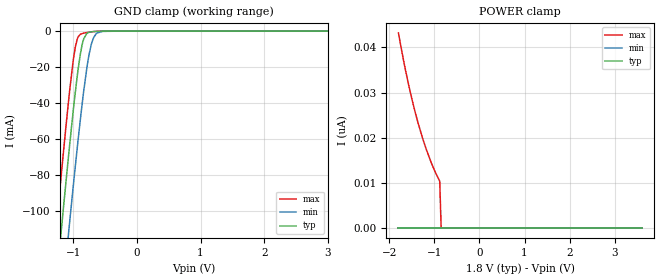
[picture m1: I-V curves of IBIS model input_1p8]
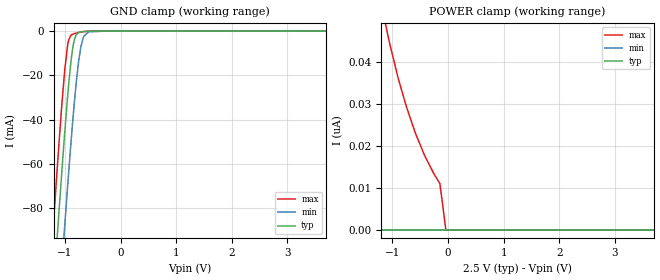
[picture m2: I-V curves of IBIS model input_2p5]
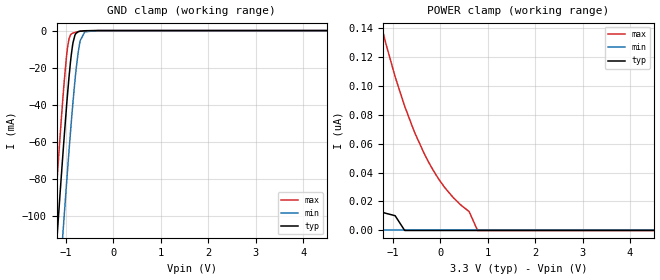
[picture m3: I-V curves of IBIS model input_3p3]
|Texas Instruments Incorporated
| Single Power Supply Single Buffer GATE with 3-State Output CMOS Logic
| Level Shifter
| Marketing part#   Digital Voltage Range   Package-type   #pins
| SN74LV4T125PWR   1.6V-5.5V   TSSOP   14
| SN74LV4T125RGYR   1.6V-5.5V   VQFN   14
[IBIS Ver]   4.1
[File name]   sn74lv4t125.ibs
[File Rev]   1.0
[Date]   3/20/2014
[Source]   Model built from TISPICE simulations at:
   Texas Instruments Incorporated.
   Analog-eLab, HPA
   12500 TI Blvd
   Dallas, TX -75243
   For Support e-mail: elab_ibis@list.ti.com
[Notes]   Revision History:
   Rev 1.0: 3/20/2014
   - Initial model based single channel device SN74LV1T125.
   - Model generated from simulations in TISPICE
   - Model matched to SPICE simulation
   - C_comp although listed in numerical order of value are
   obtained from varying PVT conditions. For PVT conditions for
   each specific value refer the buffer description under
   respective [Model]. IBIS model user is responsible for using
   appropriate C_comp to simulate for Signal Integrity.
[Disclaimer]
| This model is designed as an aid for customers of Texas Instruments.
| TI and its licensors and suppliers make no warranties, either expressed
| or implied, with respect to this  model, including the warranties of
| merchantability or fitness for a particular purpose. The model is
| provided solely on an "as is" basis. The entire risk as to its quality
| and performance is with the customer.
[Copyright]
(C) Copyright 2014 Texas Instruments Incorporated.All rights reserved.
|   SN74LV4T125PW
[Component]   SN74LV1T425PW
[Manufacturer]   TI
[Package]   |14 TSSOP  -  PW package
|   typ   min   max
R_pkg   0.19103   0.16967   0.21164
L_pkg   3.05250nH   2.65688nH   3.60685nH
C_pkg   0.48736pF   0.46092pF   0.53275pF
[Pin]  signal_name   model_name   R_pin   L_pin   C_pin
1   1OE   INPUT   0.19696   3.49379nH  0.52991pF
2   1A   INPUT   0.20002   3.01515nH  0.47995pF
3   1Y   OUTPUT   0.17897   2.78188nH  0.46369pF
4   2OE   INPUT   0.16967   2.65688nH  0.46092pF
5   2A   INPUT   0.17977   2.79132nH  0.46440pF
6   2Y   OUTPUT   0.19791   3.00095nH  0.47800pF
7   GND   GND   0.20476   3.55750nH  0.53043pF
8   3Y   OUTPUT   0.19575   3.49014nH  0.52950pF
9   3A   INPUT   0.20186   3.03224nH  0.48111pF
10   3OE   INPUT   0.18274   2.81298nH  0.46552pF
11   4Y   OUTPUT   0.17138   2.66909nH  0.46209pF
12   4A   INPUT   0.18361   2.81712nH  0.46577pF
13   4OE   INPUT   0.19944   3.00908nH  0.47904pF
14   VCC   POWER   0.21164   3.60685nH  0.53275pF
|   SN74LV1T125RGY
[Component]   SN74LV1T125RGY
[Manufacturer]   TI
[Package]   |14 VQFN   -  RGY package
|   typ   min   max
R_pkg   0.08979   0.08149   0.10052
L_pkg   1.30240nH   1.17387nH   1.47310nH
C_pkg   0.16924pF   0.14978pF   0.18157pF
[Pin]  signal_name   model_name   R_pin   L_pin   C_pin
1   1OE   INPUT   0.09263   1.35701nH  0.15000pF
2   1A   INPUT   0.09350   1.36263nH  0.17161pF
3   1Y   OUTPUT   0.08314   1.19921nH  0.17913pF
4   2OE   INPUT   0.08149   1.17387nH  0.17731pF
5   2A   INPUT   0.08375   1.20851nH  0.18057pF
6   2Y   OUTPUT   0.09332   1.36003nH  0.17060pF
7   GND   GND   0.09689   1.42225nH  0.15288pF
8   3Y   OUTPUT   0.09197   1.34335nH  0.14978pF
9   3A   INPUT   0.09427   1.36703nH  0.17200pF
10   3OE   INPUT   0.08447   1.21111nH  0.18075pF
11   4Y   OUTPUT   0.08222   1.17617nH  0.17808pF
12   4A   INPUT   0.08532   1.22381nH  0.18157pF
13   4OE   INPUT   0.09352   1.35553nH  0.17041pF
14   VCC   POWER   0.10052   1.47310nH  0.15470pF
|   Model Selectors
[Model Selector] INPUT
input_1p8   1.8V  digital input
input_2p5   2.5V  digital input
input_3p3   3.3V  digital input
input_5p0   5.0V  digital input
[Model Selector] OUTPUT
output_1p8   1.8V  digital 3-state
output_2p5   2.5V  digital 3-state
output_3p3   3.3V  digital 3-state
output_5p0   5.0V  digital 3-state
| Models and submodels in the file (8): input_1p8 (Input), input_2p5 (Input), input_3p3 (Input), input_5p0 (Input), output_1p8 (3-state), output_2p5 (3-state), output_3p3 (3-state), output_5p0 (3-state)
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|   input_1p8 Model
[Model]   input_1p8
Model_type   Input
Vinl = 0.57
Vinh = 0.95
|   typ   min   max
|   (nom PVT)   (fast PVT)   (slow PVT)
C_comp   6.973e-13   6.927e-13   7.020e-13
[Model spec]
|subparameter
Vinl   0.57   0.57   0.57
Vinh   0.95   0.95   0.99
| Where nom  PVT is Nominal Process, 1.8V, 40C
|   Fast PVT is Strong Process,  1.98V, -40C
|   Slow PVT is Weak Process,   1.62V, 140C
[Voltage Range]   1.8   1.62   1.98
|Junction Temperature
[Temperature Range]   40   140   -40
[Power Clamp Reference]   1.8   1.62   1.98
[GND Clamp Reference]   0   0   0
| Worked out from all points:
|   GND clamp passes 1 mA (typ) near -0.77 V on its own axis
[GND Clamp]
|   Voltage   I(typ)   I(min)   I(max)
-1.8V     -349mA     -390mA     -320.7mA
-1.4V     -191.8mA   -234.7mA   -161.5mA
-1.2V     -115.7mA   -159.1mA   -84.63mA
-1.165V   -102.5mA   -145.9mA   -71.47mA
-1.071V   -68.72mA   -111.8mA   -38.32mA
-968.4mV  -34.53mA   -75.73mA   -9.255mA
-887.4mV  -12.81mA   -49.13mA   -1.824mA
-833.4mV  -4.24mA    -33.01mA   -1.152mA
-750.2mV  -670.7uA   -12.99mA   -614.3uA
-680.6mV  -250.8uA   -3.714mA   -303.4uA
-623.9mV  -121.5uA   -1.06mA    -143.4uA
3.6V      0A         0A         0A
[POWER Clamp]
|   Voltage   I(typ)   I(min)   I(max)
-1.8V     0A         0A         43.21nA
-1.675V   0A         0A         36.55nA
-1.588V   0A         0A         32.38nA
-1.457V   0A         0A         26.8nA
-1.366V   0A         0A         23.36nA
-1.251V   0A         0A         19.51nA
-1.085V   0A         0A         14.84nA
-984.2mV  0A         0A         12.45nA
-883.1mV  0A         0A         10.37nA
-851.4mV  0A         0A         0A
3.6V      0A         0A         0A
|   input_2p5 Model
[Model]   input_2p5
Model_type   Input
Vinl = 0.75
Vinh = 1.145
|   typ   min   max
|   (nom PVT)   (fast PVT)   (slow PVT)
C_comp   6.859e-13   6.814e-13   6.904e-13
[Model spec]
|subparameter
Vinl   0.75   0.75   0.75
Vinh   1.145   1.145   1.22
| Where nom  PVT is Nominal Process, 2.5V, 40C
|   Fast PVT is Strong Process,  2.75V, -40C
|   Slow PVT is Weak Process,   2.25V, 140C
[Voltage Range]   2.5   2.25   2.75
|Junction Temperature
[Temperature Range]   40   140   -40
[Power Clamp Reference]   2.5   2.25   2.75
[GND Clamp Reference]   0   0   0
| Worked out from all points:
|   GND clamp passes 1 mA (typ) near -0.77 V on its own axis
[GND Clamp]
|   Voltage   I(typ)   I(min)   I(max)
-2.5V     -629.8mA   -667.3mA   -604.3mA
-1.232V   -127.8mA   -171.2mA   -96.85mA
-1.145V   -95.5mA    -138.9mA   -64.49mA
-1.105V   -80.81mA   -124.1mA   -50mA
-1.008V   -47.03mA   -89.23mA   -18.62mA
-943mV    -26.96mA   -67.16mA   -5.2mA
-862.5mV  -8.087mA   -41.49mA   -1.429mA
-792.3mV  -1.573mA   -22.16mA   -860.5uA
-713.5mV  -383.8uA   -7.11mA    -434.7uA
-654.8mV  -181.4uA   -2.119mA   -220.4uA
-571.7mV  -57.55uA   -335.5uA   -61.53uA
5V        0A         0A         0A
[POWER Clamp]
|   Voltage   I(typ)   I(min)   I(max)
-2.5V     17.64nA    0A         203.4nA
-1.738V   10.07nA    0A         99.15nA
-1.675V   0A         0A         92.8nA
-1.185V   0A         0A         52.7nA
-1.051V   0A         0A         44.4nA
-890mV    0A         0A         35.79nA
-748.2mV  0A         0A         29.29nA
-587.5mV  0A         0A         23.05nA
-423.8mV  0A         0A         17.78nA
-146mV    0A         0A         11.01nA
-38.75mV  0A         0A         0A
5V        0A         0A         0A
|   input_3p3 Model
[Model]   input_3p3
Model_type   Input
Vinl = 0.8
Vinh = 1.37
|   typ   min   max
|   (nom PVT)   (fast PVT)   (slow PVT)
C_comp   6.770e-13   6.726e-13   6.814e-13
[Model spec]
|subparameter
Vinl   0.8   0.8   0.8
Vinh   1.37   1.37   1.47
| Where nom  PVT is Nominal Process, 3.3V, 40C
|   Fast PVT is Strong Process,  3.6V, -40C
|   Slow PVT is Weak Process,   3V, 140C
[Voltage Range]   3.3   3   3.6
|Junction Temperature
[Temperature Range]   40   140   -40
[Power Clamp Reference]   3.3   3   3.6
[GND Clamp Reference]   0   0   0
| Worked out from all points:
|   GND clamp passes 1 mA (typ) near -0.76 V on its own axis
[GND Clamp]
|   Voltage   I(typ)   I(min)   I(max)
-3.3V     -954.2mA   -987.6mA   -931.2mA
-1.647V   -288.4mA   -330.2mA   -259.4mA
-1.252V   -135mA     -178.4mA   -104.1mA
-1.226V   -125.5mA   -168.9mA   -94.54mA
-1.126V   -88.25mA   -131.6mA   -57.31mA
-1.065V   -66.62mA   -109.6mA   -36.32mA
-966.9mV  -34.07mA   -75.22mA   -8.966mA
-861mV    -7.844mA   -41.04mA   -1.412mA
-795.3mV  -1.688mA   -22.9mA    -880.2uA
-712.8mV  -380.1uA   -7.022mA   -431.6uA
-603mV    -91.15uA   -664.8uA   -104.1uA
6.6V      0A         0A         0A
[POWER Clamp]
|   Voltage   I(typ)   I(min)   I(max)
-3.3V     46.68nA    0A         641.2nA
-2.436V   28.44nA    0A         371.7nA
-1.345V   13.71nA    0A         155.4nA
-1.171V   12.05nA    0A         132nA
-952.8mV  10.19nA    0A         106.1nA
-751.2mV  0A         0A         85.68nA
-542.4mV  0A         0A         67.68nA
-330mV    0A         0A         52.37nA
112.8mV   0A         0A         28.82nA
607.2mV   0A         0A         13.09nA
786mV     0A         0A         0A
6.6V      0A         0A         0A
